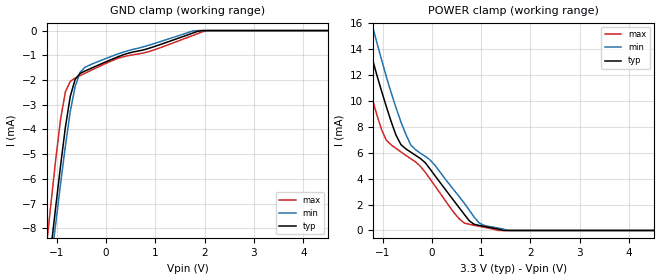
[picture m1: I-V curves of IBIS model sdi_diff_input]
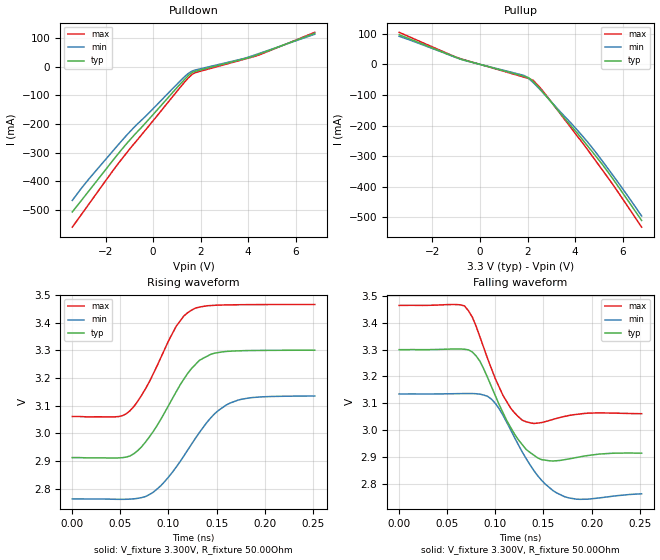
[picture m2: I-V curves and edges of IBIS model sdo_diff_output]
|   National Semiconductor Corporation
|   IBIS Model of LMH0356
[IBIS Ver]   4.2
[Comment char]  |_char
[File name]   lmh0356sq.ibs
[File Rev]   1.0
[Date]   2/4/2010
[Source]   From silicon level SPICE model of family device (lmh0344)
[Notes]   Generated by National Semiconductor Corp.
|   This model only supports the HIGH SPEED DATA PATH pins:
|   FR4 EQ is not supported in  this Model
|   Generic High Speed input model ONLY (SDIn, SDInbar)
|   CML Ouput model for SDO, SDObar, SCO/SDO2, and SCO/SDO2bar
| Begin IBIS Parser Results
| Don't edit this section manually!
Timestamp: 02/08/2010
IBISCHK5 V5.0.0
Checking lmh0356sq.ibs for IBIS 4.2
Compatibility...
Errors  : 0
File Passed
| End IBIS Parser Results
[Disclaimer]
(C) Copyright National Semiconductor Corporation 2010
   All rights reserved
   National Semiconductor Corporation hereby grants
the user of this IBIS model a non-exclusive, nontransferable
license to use this IBIS model under the following terms.
Before using this IBIS model, the user should read this
license.  If the user does not accept these terms,  the
IBIS model should be returned to National within 30 days.
   The user is granted this license only to use the
IBIS model and is not granted rights to sell, load, rent,
lease or license the IBIS model in whole or in part, or in
modified form to anyone other than user. User may modify
the IBIS model to suit its specific applications but rights
to derivative works and such modifications shall belong to
National.
   This IBIS model is provided on an "AS IS" basis and
National makes absolutely no warranty with respect to the
information contained herein.NATIONAL DISCLAIMS AND CUSTOMER
WAIVES ALL WARRANTIES, EXPRESS OR IMPLIED, INCLUDING
WARRANTIES OF MERCHANTABILITY OR FITNESS FOR A PARTICULAR
PURPOSE. The entire risk as to quality and performance is
with the Customer. ACCORDINGLY, IN NO EVENT SHALL THE
COMPANY BE LIABLE FOR ANY DAMAGES, WHETHER IN CONTRACT OR
TORT,INCLUDING ANY LOST PROFITS OR OTHER INCIDENTAL,
CONSEQUENTIAL, EXEMPLARY, OR PUNITIVE DAMAGES ARISING OUT
OF THE USE OR APPLICATION OF THE IBIS model provided in
this package.Further, National reserves the right to make
changes without notice to any product herein to improve
reliability, function, or design. National does not convey
any license under patent rights or any other intellectual
property rights, including those of third parties.
   National is not obligated to provide maintenance or support
for the licensed IBIS model.
[Component]   LMH0356
[Manufacturer]  National Semiconductor
[Package]
|   typ   min   max
R_pkg   0   0   0
L_pkg   0   0   0
C_pkg   0   0   0
[PIN]   signal_name   model_name   R_pin   L_pin   C_pin
1   SDI0   sdi_diff_input
2   SDI0b   sdi_diff_input
3   VCC   POWER
4   SDI1   sdi_diff_input
5   SDI1b   sdi_diff_input
6   VCC   POWER
7   SDI2   sdi_diff_input
8   SDI2b   sdi_diff_input
9   ENABLE   NC
10   SDI3   sdi_diff_input
11   SDI3b   sdi_diff_input
12   VCC   POWER
13   VEE   GND
14   VCC   POWER
15   BYPASS   NC
16   MUTEb   NC
17   VEE   GND
18   XTALin   NC
19   VEE   GND
20   VEE   GND
21   VEE   GND
22   XTALout   NC
23   VEE   GND
24   LOCK   NC
25   VEE   GND
26   VEE   GND
27   VEE   GND
28   SCO/SDO2b   sdo_diff_output
29   SCO/SCO2   sdo_diff_output
30   VCC   POWER
31   VCC   POWER
32   SDOb   sdo_diff_output
33   SDO   sdo_diff_output
34   VCC   POWER
35   VCC   POWER
36   SD/HDb   NC
37   SCOEN   NC
38   VEE   GND
39   VEE   GND
40   VEE   GND
41   VEE   GND
42   VEE   GND
43   LF1   NC
44   LF2   NC
45   RATE0   NC
46   RATE1   NC
47   SEL0   NC
48   SEL1   NC
49   DAP   GND
[Diff_pin]   inv_pin   vdiff   tdelay_typ   tdelay_min   tdelay_max
| The '+' pin is Diff_pin and the '-' pin is the inv_pin
1   2   0.050   0 0 0
4   5   0.050   0 0 0
7   8   0.050   0 0 0
10   11   0.050   0 0 0
29   28   0.000   0 0 0
33   32   0.000   0 0 0
[Package Model]  48 LLP for LMH0356
|   Package Model
[Define Package Model]  48 LLP for LMH0356
[Manufacturer]  National Semiconductor
[OEM] NA
[Description]  Package Model for LMH0356
[Number Of Pins]  49
[Pin Numbers]
49   | 49 = DAP
1   | 1 = L1
2   | 2 = L2
3   | 3 = L3
4   | 4 = L4
5   | 5 = L5
6   | 6 = L6
7   | 7 = L7
8   | 8 = L8
9   | 9 = L9
10   | 10 = L10
11   | 11 = L11
12   | 12 = L12
13   | 13 = L13
14   | 14 = L14
15   | 15 = L15
16   | 16 = L16
17   | 17 = L17
18   | 18 = L18
19   | 19 = L19
20   | 20 = L20
21   | 21 = L21
22   | 22 = L22
23   | 23 = L23
24   | 24 = L24
25   | 25 = L25
26   | 26 = L26
27   | 27 = L27
28   | 28 = L28
29   | 29 = L29
30   | 30 = L30
31   | 31 = L31
32   | 32 = L32
33   | 33 = L33
34   | 34 = L34
35   | 35 = L35
36   | 36 = L36
37   | 37 = L37
38   | 38 = L38
39   | 39 = L39
40   | 40 = L40
41   | 41 = L41
42   | 42 = L42
43   | 43 = L43
44   | 44 = L44
45   | 45 = L45
46   | 46 = L46
47   | 47 = L47
48   | 48 = L48
[Model Data]
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[End Model Data]
[End Package Model]
| Models and submodels in the file (2): sdi_diff_input (Input), sdo_diff_output (Output)
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[Model]   sdi_diff_input
Model_type   Input
| Differential Input thresholds are +/- 50mV differential
| [Diff_pin] over rides Vinl/Vinh when used differentially
Vinl=0.8V
Vinh=2.0V
|   typ   min   max
C_comp   2.100pF   2.000pF   2.200pF
[Voltage Range]   3.300V   3.135   3.465
[Temperature Range]   25.0   85.0   -40.0
[GND Clamp]
|Voltage   I(typ)   I(min)   I(max)
-3.399V   -53.67mA   -52.93mA   -53.54mA
-1.221V   -10.64mA   -11.17mA   -8.938mA
-1.122V   -8.892mA   -9.492mA   -7.072mA
-1.023V   -7.168mA   -7.84mA    -5.255mA
-924mV    -5.487mA   -6.223mA   -3.607mA
-825mV    -3.913mA   -4.669mA   -2.476mA
-726mV    -2.66mA    -3.271mA   -2.056mA
-627mV    -1.977mA   -2.265mA   -1.923mA
-528mV    -1.735mA   -1.694mA   -1.825mA
-132mV    -1.376mA   -1.231mA   -1.447mA
2.046V    0A         0A         0A
6.798V    0A         0A         0A
[Power Clamp]
|Voltage   I(typ)   I(min)   I(max)
-3.399V   97.59mA    109.5mA    86.47mA
-1.617V   19.58mA    24.39mA    16.35mA
-1.419V   16.45mA    19.33mA    13.16mA
-1.221V   13.46mA    16.03mA    10.34mA
-924mV    9.577mA    11.89mA    6.977mA
-627mV    6.634mA    8.376mA    6.072mA
-429mV    6.055mA    6.614mA    5.552mA
-132mV    5.227mA    5.731mA    4.484mA
660mV     1.231mA    2.096mA    566.7uA
957mV     391.4uA    588.8uA    326.6uA
1.551V    0A         0A         0A
6.798V    0A         0A         0A
[Model]   sdo_diff_output
Model_type   Output
Vmeas = 3.1V   | Single-Ended Crossing Point for SDO and SDOb
Vref = 3.3V
Cref = 0.000F
Rref = 50.000Ohm
|   typ   min   max
C_comp   0.700pF   0.600pF   0.800pF
[Voltage Range]   3.300V   3.135   3.465
[Temperature Range]   25.0   85.0   -40.0
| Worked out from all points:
|   slope of the pulldown table from 0 to 0.495 V, typ, clamps not added: 10.7 ohm
|   slope of the pullup table from 0 to 0.495 V, typ, clamps not added: 47.5 ohm
|   falling waveform, V_fixture 3.300V, R_fixture 50.00Ohm: 20-80 % time 30.4ps typ, 35.4ps min, 26ps max; typ from 3.3 V to 2.91 V
|   rising waveform, V_fixture 3.300V, R_fixture 50.00Ohm: 20-80 % time 40.6ps typ, 46.2ps min, 34.9ps max; typ from 2.91 V to 3.3 V
[Pullup]
|Voltage   I(typ)   I(min)   I(max)
-3.399V   97mA       91.63mA    104.8mA
-924mV    20.55mA    19.83mA    21.22mA
1.848V    -38.91mA   -36.34mA   -41.8mA
2.046V    -43.79mA   -46.16mA   -46.28mA
2.244V    -57.09mA   -59.86mA   -52.34mA
2.739V    -99.43mA   -100.4mA   -96.51mA
3.828V    -201.1mA   -192mA     -207.5mA
4.62V     -275.7mA   -262.8mA   -289mA
5.412V    -355.1mA   -343.8mA   -373.8mA
6.798V    -510.4mA   -495.8mA   -532.3mA
[Pulldown]
|Voltage   I(typ)   I(min)   I(max)
-3.399V   -506mA     -466mA     -559mA
-2.706V   -433.5mA   -391.9mA   -479.3mA
-1.716V   -329.3mA   -296.2mA   -365.4mA
-1.023V   -259.8mA   -231mA     -291mA
1.254V    -50.98mA   -40.73mA   -61.01mA
1.452V    -33.68mA   -25.81mA   -42.01mA
1.65V     -20.41mA   -15.26mA   -26.64mA
1.848V    -14.67mA   -10.43mA   -19.38mA
3.828V    27.07mA    28.39mA    25.48mA
4.323V    39.26mA    41.71mA    36.69mA
6.798V    115.9mA    112.6mA    119.2mA
[Ramp]
R_load = 50.00Ohm
|   typ   min   max
dV/dt_r   0.24/43p   0.225/47p   0.25/38p
dV/dt_f   0.24/31p   0.225/37p   0.25/28p
[Falling Waveform]
V_fixture = 3.300V
V_fixture_min = 3.135V
V_fixture_max = 3.465V
R_fixture = 50.00Ohm
|Time   V(typ)   V(min)   V(max)
0s        3.3V       3.135V     3.465V
68ps      3.301V     3.136V     3.463V
76ps      3.292V     3.136V     3.422V
84ps      3.257V     3.134V     3.347V
96ps      3.161V     3.115V     3.228V
108ps     3.064V     3.055V     3.129V
128ps     2.946V     2.918V     3.037V
148ps     2.89V      2.813V     3.028V
172ps     2.89V      2.752V     3.051V
252ps     2.914V     2.763V     3.061V
[Rising Waveform]
V_fixture = 3.300V
V_fixture_min = 3.135V
V_fixture_max = 3.465V
R_fixture = 50.00Ohm
|Time   V(typ)   V(min)   V(max)
0s        2.912V     2.763V     3.061V
48ps      2.911V     2.762V     3.061V
60ps      2.918V     2.763V     3.082V
76ps      2.968V     2.772V     3.16V
92ps      3.051V     2.811V     3.273V
108ps     3.15V      2.878V     3.387V
128ps     3.249V     2.982V     3.452V
148ps     3.29V      3.071V     3.462V
172ps     3.298V     3.12V      3.464V
252ps     3.3V       3.135V     3.465V
